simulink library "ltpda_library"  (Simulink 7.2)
settings: Solver=ode45  SolverMode=SingleTasking  StartTime=0.0  StopTime=10.0  RelTol=1e-3
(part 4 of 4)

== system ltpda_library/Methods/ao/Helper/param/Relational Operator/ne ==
  In1 : Inport  OutDataType=sfix(16)  OutScaling=2^0
  ne : M-S-Function  Tag=ne  FunctionName=ltpdasim
  Out1 : Outport  OutDataType=sfix(16)  OutScaling=2^0
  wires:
  In1/1 -> ne/1
  ne/1 -> Out1/1

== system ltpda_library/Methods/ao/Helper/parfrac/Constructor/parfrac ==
  Ground : Ground
  parfrac : M-S-Function  Tag=parfrac  FunctionName=ltpdasim
  Out1 : Outport  OutDataType=sfix(16)  OutScaling=2^0
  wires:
  Ground/1 -> parfrac/1
  parfrac/1 -> Out1/1

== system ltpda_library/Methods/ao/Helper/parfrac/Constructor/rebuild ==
  Ground : Ground
  rebuild : M-S-Function  Tag=rebuild  FunctionName=ltpdasim
  Out1 : Outport  OutDataType=sfix(16)  OutScaling=2^0
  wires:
  Ground/1 -> rebuild/1
  rebuild/1 -> Out1/1

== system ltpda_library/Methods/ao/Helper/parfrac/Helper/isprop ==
  In1 : Inport  OutDataType=sfix(16)  OutScaling=2^0
  isprop : M-S-Function  Tag=isprop  FunctionName=ltpdasim
  Out1 : Outport  OutDataType=sfix(16)  OutScaling=2^0
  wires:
  In1/1 -> isprop/1
  isprop/1 -> Out1/1

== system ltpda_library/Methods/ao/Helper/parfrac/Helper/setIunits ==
  In1 : Inport  OutDataType=sfix(16)  OutScaling=2^0
  setIunits : M-S-Function  Tag=setIunits  FunctionName=ltpdasim
  Out1 : Outport  OutDataType=sfix(16)  OutScaling=2^0
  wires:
  In1/1 -> setIunits/1
  setIunits/1 -> Out1/1

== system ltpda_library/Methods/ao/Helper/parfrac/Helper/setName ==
  In1 : Inport  OutDataType=sfix(16)  OutScaling=2^0
  setName : M-S-Function  Tag=setName  FunctionName=ltpdasim
  Out1 : Outport  OutDataType=sfix(16)  OutScaling=2^0
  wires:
  In1/1 -> setName/1
  setName/1 -> Out1/1

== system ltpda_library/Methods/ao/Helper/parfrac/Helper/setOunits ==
  In1 : Inport  OutDataType=sfix(16)  OutScaling=2^0
  setOunits : M-S-Function  Tag=setOunits  FunctionName=ltpdasim
  Out1 : Outport  OutDataType=sfix(16)  OutScaling=2^0
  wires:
  In1/1 -> setOunits/1
  setOunits/1 -> Out1/1

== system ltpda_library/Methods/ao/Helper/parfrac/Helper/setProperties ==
  In1 : Inport  OutDataType=sfix(16)  OutScaling=2^0
  setProperties : M-S-Function  Tag=setProperties  FunctionName=ltpdasim
  Out1 : Outport  OutDataType=sfix(16)  OutScaling=2^0
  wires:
  In1/1 -> setProperties/1
  setProperties/1 -> Out1/1

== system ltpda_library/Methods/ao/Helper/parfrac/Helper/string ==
  In1 : Inport  OutDataType=sfix(16)  OutScaling=2^0
  string : M-S-Function  Tag=string  FunctionName=ltpdasim
  Out1 : Outport  OutDataType=sfix(16)  OutScaling=2^0
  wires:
  In1/1 -> string/1
  string/1 -> Out1/1

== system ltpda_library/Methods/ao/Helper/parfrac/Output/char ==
  In1 : Inport  OutDataType=sfix(16)  OutScaling=2^0
  Terminator : Terminator
  char : M-S-Function  Tag=char  FunctionName=ltpdasim
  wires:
  char/1 -> Terminator/1
  In1/1 -> char/1

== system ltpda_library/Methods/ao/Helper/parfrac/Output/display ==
  In1 : Inport  OutDataType=sfix(16)  OutScaling=2^0
  Terminator : Terminator
  display : M-S-Function  Tag=display  FunctionName=ltpdasim
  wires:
  display/1 -> Terminator/1
  In1/1 -> display/1

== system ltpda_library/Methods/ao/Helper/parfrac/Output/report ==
  In1 : Inport  OutDataType=sfix(16)  OutScaling=2^0
  Terminator : Terminator
  report : M-S-Function  Tag=report  FunctionName=ltpdasim
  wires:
  report/1 -> Terminator/1
  In1/1 -> report/1

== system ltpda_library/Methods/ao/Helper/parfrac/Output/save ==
  In1 : Inport  OutDataType=sfix(16)  OutScaling=2^0
  Terminator : Terminator
  save : M-S-Function  Tag=save  FunctionName=ltpdasim
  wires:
  save/1 -> Terminator/1
  In1/1 -> save/1

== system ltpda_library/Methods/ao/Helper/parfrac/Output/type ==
  In1 : Inport  OutDataType=sfix(16)  OutScaling=2^0
  Terminator : Terminator
  type : M-S-Function  Tag=type  FunctionName=ltpdasim
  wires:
  type/1 -> Terminator/1
  In1/1 -> type/1

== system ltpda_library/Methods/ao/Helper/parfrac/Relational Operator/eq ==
  In1 : Inport  OutDataType=sfix(16)  OutScaling=2^0
  eq : M-S-Function  Tag=eq  FunctionName=ltpdasim
  Out1 : Outport  OutDataType=sfix(16)  OutScaling=2^0
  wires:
  In1/1 -> eq/1
  eq/1 -> Out1/1

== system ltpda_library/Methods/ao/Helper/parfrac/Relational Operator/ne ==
  In1 : Inport  OutDataType=sfix(16)  OutScaling=2^0
  ne : M-S-Function  Tag=ne  FunctionName=ltpdasim
  Out1 : Outport  OutDataType=sfix(16)  OutScaling=2^0
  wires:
  In1/1 -> ne/1
  ne/1 -> Out1/1

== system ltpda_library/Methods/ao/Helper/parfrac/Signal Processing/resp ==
  In1 : Inport  OutDataType=sfix(16)  OutScaling=2^0
  resp : M-S-Function  Tag=resp  FunctionName=ltpdasim
  Out1 : Outport  OutDataType=sfix(16)  OutScaling=2^0
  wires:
  In1/1 -> resp/1
  resp/1 -> Out1/1

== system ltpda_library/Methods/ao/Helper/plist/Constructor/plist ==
  Ground : Ground
  plist : M-S-Function  Tag=plist  FunctionName=ltpdasim
  Out1 : Outport  OutDataType=sfix(16)  OutScaling=2^0
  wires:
  Ground/1 -> plist/1
  plist/1 -> Out1/1

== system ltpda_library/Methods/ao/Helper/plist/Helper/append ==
  In1 : Inport  OutDataType=sfix(16)  OutScaling=2^0
  append : M-S-Function  Tag=append  FunctionName=ltpdasim
  Out1 : Outport  OutDataType=sfix(16)  OutScaling=2^0
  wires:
  In1/1 -> append/1
  append/1 -> Out1/1

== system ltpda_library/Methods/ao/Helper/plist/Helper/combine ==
  In1 : Inport  OutDataType=sfix(16)  OutScaling=2^0
  combine : M-S-Function  Tag=combine  FunctionName=ltpdasim
  Out1 : Outport  OutDataType=sfix(16)  OutScaling=2^0
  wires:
  In1/1 -> combine/1
  combine/1 -> Out1/1

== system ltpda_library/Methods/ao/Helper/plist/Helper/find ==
  In1 : Inport  OutDataType=sfix(16)  OutScaling=2^0
  find : M-S-Function  Tag=find  FunctionName=ltpdasim
  Out1 : Outport  OutDataType=sfix(16)  OutScaling=2^0
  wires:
  In1/1 -> find/1
  find/1 -> Out1/1

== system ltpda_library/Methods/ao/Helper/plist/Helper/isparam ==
  In1 : Inport  OutDataType=sfix(16)  OutScaling=2^0
  isparam : M-S-Function  Tag=isparam  FunctionName=ltpdasim
  Out1 : Outport  OutDataType=sfix(16)  OutScaling=2^0
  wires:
  In1/1 -> isparam/1
  isparam/1 -> Out1/1

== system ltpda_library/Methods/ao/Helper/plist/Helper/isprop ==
  In1 : Inport  OutDataType=sfix(16)  OutScaling=2^0
  isprop : M-S-Function  Tag=isprop  FunctionName=ltpdasim
  Out1 : Outport  OutDataType=sfix(16)  OutScaling=2^0
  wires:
  In1/1 -> isprop/1
  isprop/1 -> Out1/1

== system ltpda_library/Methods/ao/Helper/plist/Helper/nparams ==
  In1 : Inport  OutDataType=sfix(16)  OutScaling=2^0
  nparams : M-S-Function  Tag=nparams  FunctionName=ltpdasim
  Out1 : Outport  OutDataType=sfix(16)  OutScaling=2^0
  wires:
  In1/1 -> nparams/1
  nparams/1 -> Out1/1

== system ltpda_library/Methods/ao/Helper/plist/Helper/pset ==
  In1 : Inport  OutDataType=sfix(16)  OutScaling=2^0
  pset : M-S-Function  Tag=pset  FunctionName=ltpdasim
  Out1 : Outport  OutDataType=sfix(16)  OutScaling=2^0
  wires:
  In1/1 -> pset/1
  pset/1 -> Out1/1

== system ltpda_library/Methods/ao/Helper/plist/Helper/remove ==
  In1 : Inport  OutDataType=sfix(16)  OutScaling=2^0
  remove : M-S-Function  Tag=remove  FunctionName=ltpdasim
  Out1 : Outport  OutDataType=sfix(16)  OutScaling=2^0
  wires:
  In1/1 -> remove/1
  remove/1 -> Out1/1

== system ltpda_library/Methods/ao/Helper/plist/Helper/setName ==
  In1 : Inport  OutDataType=sfix(16)  OutScaling=2^0
  setName : M-S-Function  Tag=setName  FunctionName=ltpdasim
  Out1 : Outport  OutDataType=sfix(16)  OutScaling=2^0
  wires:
  In1/1 -> setName/1
  setName/1 -> Out1/1

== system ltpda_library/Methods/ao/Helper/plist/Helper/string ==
  In1 : Inport  OutDataType=sfix(16)  OutScaling=2^0
  string : M-S-Function  Tag=string  FunctionName=ltpdasim
  Out1 : Outport  OutDataType=sfix(16)  OutScaling=2^0
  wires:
  In1/1 -> string/1
  string/1 -> Out1/1

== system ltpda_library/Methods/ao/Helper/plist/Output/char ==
  In1 : Inport  OutDataType=sfix(16)  OutScaling=2^0
  Terminator : Terminator
  char : M-S-Function  Tag=char  FunctionName=ltpdasim
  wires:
  char/1 -> Terminator/1
  In1/1 -> char/1

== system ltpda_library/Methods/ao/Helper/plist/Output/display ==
  In1 : Inport  OutDataType=sfix(16)  OutScaling=2^0
  Terminator : Terminator
  display : M-S-Function  Tag=display  FunctionName=ltpdasim
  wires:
  display/1 -> Terminator/1
  In1/1 -> display/1

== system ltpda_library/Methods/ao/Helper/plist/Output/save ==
  In1 : Inport  OutDataType=sfix(16)  OutScaling=2^0
  Terminator : Terminator
  save : M-S-Function  Tag=save  FunctionName=ltpdasim
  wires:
  save/1 -> Terminator/1
  In1/1 -> save/1

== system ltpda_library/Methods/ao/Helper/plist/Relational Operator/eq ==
  In1 : Inport  OutDataType=sfix(16)  OutScaling=2^0
  eq : M-S-Function  Tag=eq  FunctionName=ltpdasim
  Out1 : Outport  OutDataType=sfix(16)  OutScaling=2^0
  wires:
  In1/1 -> eq/1
  eq/1 -> Out1/1

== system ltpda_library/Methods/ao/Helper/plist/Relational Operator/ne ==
  In1 : Inport  OutDataType=sfix(16)  OutScaling=2^0
  ne : M-S-Function  Tag=ne  FunctionName=ltpdasim
  Out1 : Outport  OutDataType=sfix(16)  OutScaling=2^0
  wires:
  In1/1 -> ne/1
  ne/1 -> Out1/1

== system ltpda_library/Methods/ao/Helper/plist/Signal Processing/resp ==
  In1 : Inport  OutDataType=sfix(16)  OutScaling=2^0
  resp : M-S-Function  Tag=resp  FunctionName=ltpdasim
  Out1 : Outport  OutDataType=sfix(16)  OutScaling=2^0
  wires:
  In1/1 -> resp/1
  resp/1 -> Out1/1

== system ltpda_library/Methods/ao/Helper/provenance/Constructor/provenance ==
  Ground : Ground
  provenance : M-S-Function  Tag=provenance  FunctionName=ltpdasim
  Out1 : Outport  OutDataType=sfix(16)  OutScaling=2^0
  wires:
  Ground/1 -> provenance/1
  provenance/1 -> Out1/1

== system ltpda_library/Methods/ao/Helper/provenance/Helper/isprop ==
  In1 : Inport  OutDataType=sfix(16)  OutScaling=2^0
  isprop : M-S-Function  Tag=isprop  FunctionName=ltpdasim
  Out1 : Outport  OutDataType=sfix(16)  OutScaling=2^0
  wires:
  In1/1 -> isprop/1
  isprop/1 -> Out1/1

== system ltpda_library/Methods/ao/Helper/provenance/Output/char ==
  In1 : Inport  OutDataType=sfix(16)  OutScaling=2^0
  Terminator : Terminator
  char : M-S-Function  Tag=char  FunctionName=ltpdasim
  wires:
  char/1 -> Terminator/1
  In1/1 -> char/1

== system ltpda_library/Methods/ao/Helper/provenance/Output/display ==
  In1 : Inport  OutDataType=sfix(16)  OutScaling=2^0
  Terminator : Terminator
  display : M-S-Function  Tag=display  FunctionName=ltpdasim
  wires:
  display/1 -> Terminator/1
  In1/1 -> display/1

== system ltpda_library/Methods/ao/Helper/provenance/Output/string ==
  In1 : Inport  OutDataType=sfix(16)  OutScaling=2^0
  Terminator : Terminator
  string : M-S-Function  Tag=string  FunctionName=ltpdasim
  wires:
  string/1 -> Terminator/1
  In1/1 -> string/1

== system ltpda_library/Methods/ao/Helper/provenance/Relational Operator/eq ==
  In1 : Inport  OutDataType=sfix(16)  OutScaling=2^0
  eq : M-S-Function  Tag=eq  FunctionName=ltpdasim
  Out1 : Outport  OutDataType=sfix(16)  OutScaling=2^0
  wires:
  In1/1 -> eq/1
  eq/1 -> Out1/1

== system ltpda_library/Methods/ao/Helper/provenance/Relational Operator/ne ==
  In1 : Inport  OutDataType=sfix(16)  OutScaling=2^0
  ne : M-S-Function  Tag=ne  FunctionName=ltpdasim
  Out1 : Outport  OutDataType=sfix(16)  OutScaling=2^0
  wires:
  In1/1 -> ne/1
  ne/1 -> Out1/1

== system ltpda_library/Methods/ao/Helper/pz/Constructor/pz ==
  Ground : Ground
  pz : M-S-Function  Tag=pz  FunctionName=ltpdasim
  Out1 : Outport  OutDataType=sfix(16)  OutScaling=2^0
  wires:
  Ground/1 -> pz/1
  pz/1 -> Out1/1

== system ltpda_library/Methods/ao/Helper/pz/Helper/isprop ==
  In1 : Inport  OutDataType=sfix(16)  OutScaling=2^0
  isprop : M-S-Function  Tag=isprop  FunctionName=ltpdasim
  Out1 : Outport  OutDataType=sfix(16)  OutScaling=2^0
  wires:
  In1/1 -> isprop/1
  isprop/1 -> Out1/1

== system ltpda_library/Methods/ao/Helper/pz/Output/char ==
  In1 : Inport  OutDataType=sfix(16)  OutScaling=2^0
  Terminator : Terminator
  char : M-S-Function  Tag=char  FunctionName=ltpdasim
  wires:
  char/1 -> Terminator/1
  In1/1 -> char/1

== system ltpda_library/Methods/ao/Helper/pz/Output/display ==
  In1 : Inport  OutDataType=sfix(16)  OutScaling=2^0
  Terminator : Terminator
  display : M-S-Function  Tag=display  FunctionName=ltpdasim
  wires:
  display/1 -> Terminator/1
  In1/1 -> display/1

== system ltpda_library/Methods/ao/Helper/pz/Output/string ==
  In1 : Inport  OutDataType=sfix(16)  OutScaling=2^0
  Terminator : Terminator
  string : M-S-Function  Tag=string  FunctionName=ltpdasim
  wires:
  string/1 -> Terminator/1
  In1/1 -> string/1

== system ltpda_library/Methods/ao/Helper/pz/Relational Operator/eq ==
  In1 : Inport  OutDataType=sfix(16)  OutScaling=2^0
  eq : M-S-Function  Tag=eq  FunctionName=ltpdasim
  Out1 : Outport  OutDataType=sfix(16)  OutScaling=2^0
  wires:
  In1/1 -> eq/1
  eq/1 -> Out1/1

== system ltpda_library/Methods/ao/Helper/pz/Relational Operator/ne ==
  In1 : Inport  OutDataType=sfix(16)  OutScaling=2^0
  ne : M-S-Function  Tag=ne  FunctionName=ltpdasim
  Out1 : Outport  OutDataType=sfix(16)  OutScaling=2^0
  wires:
  In1/1 -> ne/1
  ne/1 -> Out1/1

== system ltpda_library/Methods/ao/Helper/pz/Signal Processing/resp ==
  In1 : Inport  OutDataType=sfix(16)  OutScaling=2^0
  resp : M-S-Function  Tag=resp  FunctionName=ltpdasim
  Out1 : Outport  OutDataType=sfix(16)  OutScaling=2^0
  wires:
  In1/1 -> resp/1
  resp/1 -> Out1/1

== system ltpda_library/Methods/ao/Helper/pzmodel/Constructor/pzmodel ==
  Ground : Ground
  pzmodel : M-S-Function  Tag=pzmodel  FunctionName=ltpdasim
  Out1 : Outport  OutDataType=sfix(16)  OutScaling=2^0
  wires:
  Ground/1 -> pzmodel/1
  pzmodel/1 -> Out1/1

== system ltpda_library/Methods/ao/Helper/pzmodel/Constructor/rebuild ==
  Ground : Ground
  rebuild : M-S-Function  Tag=rebuild  FunctionName=ltpdasim
  Out1 : Outport  OutDataType=sfix(16)  OutScaling=2^0
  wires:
  Ground/1 -> rebuild/1
  rebuild/1 -> Out1/1

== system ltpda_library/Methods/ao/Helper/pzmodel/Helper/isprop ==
  In1 : Inport  OutDataType=sfix(16)  OutScaling=2^0
  isprop : M-S-Function  Tag=isprop  FunctionName=ltpdasim
  Out1 : Outport  OutDataType=sfix(16)  OutScaling=2^0
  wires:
  In1/1 -> isprop/1
  isprop/1 -> Out1/1

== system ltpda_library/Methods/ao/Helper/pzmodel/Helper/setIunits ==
  In1 : Inport  OutDataType=sfix(16)  OutScaling=2^0
  setIunits : M-S-Function  Tag=setIunits  FunctionName=ltpdasim
  Out1 : Outport  OutDataType=sfix(16)  OutScaling=2^0
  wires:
  In1/1 -> setIunits/1
  setIunits/1 -> Out1/1

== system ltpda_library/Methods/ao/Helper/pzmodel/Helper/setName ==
  In1 : Inport  OutDataType=sfix(16)  OutScaling=2^0
  setName : M-S-Function  Tag=setName  FunctionName=ltpdasim
  Out1 : Outport  OutDataType=sfix(16)  OutScaling=2^0
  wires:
  In1/1 -> setName/1
  setName/1 -> Out1/1

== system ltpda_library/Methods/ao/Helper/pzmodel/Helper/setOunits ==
  In1 : Inport  OutDataType=sfix(16)  OutScaling=2^0
  setOunits : M-S-Function  Tag=setOunits  FunctionName=ltpdasim
  Out1 : Outport  OutDataType=sfix(16)  OutScaling=2^0
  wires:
  In1/1 -> setOunits/1
  setOunits/1 -> Out1/1

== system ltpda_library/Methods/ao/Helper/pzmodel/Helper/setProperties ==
  In1 : Inport  OutDataType=sfix(16)  OutScaling=2^0
  setProperties : M-S-Function  Tag=setProperties  FunctionName=ltpdasim
  Out1 : Outport  OutDataType=sfix(16)  OutScaling=2^0
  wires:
  In1/1 -> setProperties/1
  setProperties/1 -> Out1/1

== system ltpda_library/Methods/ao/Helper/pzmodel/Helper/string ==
  In1 : Inport  OutDataType=sfix(16)  OutScaling=2^0
  string : M-S-Function  Tag=string  FunctionName=ltpdasim
  Out1 : Outport  OutDataType=sfix(16)  OutScaling=2^0
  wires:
  In1/1 -> string/1
  string/1 -> Out1/1

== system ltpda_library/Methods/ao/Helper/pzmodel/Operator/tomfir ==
  In1 : Inport  OutDataType=sfix(16)  OutScaling=2^0
  tomfir : M-S-Function  Tag=tomfir  FunctionName=ltpdasim
  Out1 : Outport  OutDataType=sfix(16)  OutScaling=2^0
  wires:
  In1/1 -> tomfir/1
  tomfir/1 -> Out1/1

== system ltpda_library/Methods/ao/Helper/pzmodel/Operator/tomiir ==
  In1 : Inport  OutDataType=sfix(16)  OutScaling=2^0
  tomiir : M-S-Function  Tag=tomiir  FunctionName=ltpdasim
  Out1 : Outport  OutDataType=sfix(16)  OutScaling=2^0
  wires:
  In1/1 -> tomiir/1
  tomiir/1 -> Out1/1

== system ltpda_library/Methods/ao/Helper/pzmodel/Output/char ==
  In1 : Inport  OutDataType=sfix(16)  OutScaling=2^0
  Terminator : Terminator
  char : M-S-Function  Tag=char  FunctionName=ltpdasim
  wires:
  char/1 -> Terminator/1
  In1/1 -> char/1

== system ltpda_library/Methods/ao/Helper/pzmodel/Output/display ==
  In1 : Inport  OutDataType=sfix(16)  OutScaling=2^0
  Terminator : Terminator
  display : M-S-Function  Tag=display  FunctionName=ltpdasim
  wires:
  display/1 -> Terminator/1
  In1/1 -> display/1

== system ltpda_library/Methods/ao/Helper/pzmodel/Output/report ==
  In1 : Inport  OutDataType=sfix(16)  OutScaling=2^0
  Terminator : Terminator
  report : M-S-Function  Tag=report  FunctionName=ltpdasim
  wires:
  report/1 -> Terminator/1
  In1/1 -> report/1

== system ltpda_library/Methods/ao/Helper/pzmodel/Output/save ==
  In1 : Inport  OutDataType=sfix(16)  OutScaling=2^0
  Terminator : Terminator
  save : M-S-Function  Tag=save  FunctionName=ltpdasim
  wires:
  save/1 -> Terminator/1
  In1/1 -> save/1

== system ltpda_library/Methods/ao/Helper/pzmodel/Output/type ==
  In1 : Inport  OutDataType=sfix(16)  OutScaling=2^0
  Terminator : Terminator
  type : M-S-Function  Tag=type  FunctionName=ltpdasim
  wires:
  type/1 -> Terminator/1
  In1/1 -> type/1

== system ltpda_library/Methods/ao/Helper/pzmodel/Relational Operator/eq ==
  In1 : Inport  OutDataType=sfix(16)  OutScaling=2^0
  eq : M-S-Function  Tag=eq  FunctionName=ltpdasim
  Out1 : Outport  OutDataType=sfix(16)  OutScaling=2^0
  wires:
  In1/1 -> eq/1
  eq/1 -> Out1/1

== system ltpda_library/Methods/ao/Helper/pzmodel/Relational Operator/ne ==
  In1 : Inport  OutDataType=sfix(16)  OutScaling=2^0
  ne : M-S-Function  Tag=ne  FunctionName=ltpdasim
  Out1 : Outport  OutDataType=sfix(16)  OutScaling=2^0
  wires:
  In1/1 -> ne/1
  ne/1 -> Out1/1

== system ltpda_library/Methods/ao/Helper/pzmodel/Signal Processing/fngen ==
  In1 : Inport  OutDataType=sfix(16)  OutScaling=2^0
  fngen : M-S-Function  Tag=fngen  FunctionName=ltpdasim
  Out1 : Outport  OutDataType=sfix(16)  OutScaling=2^0
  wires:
  In1/1 -> fngen/1
  fngen/1 -> Out1/1

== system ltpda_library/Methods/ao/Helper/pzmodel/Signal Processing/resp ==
  In1 : Inport  OutDataType=sfix(16)  OutScaling=2^0
  resp : M-S-Function  Tag=resp  FunctionName=ltpdasim
  Out1 : Outport  OutDataType=sfix(16)  OutScaling=2^0
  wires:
  In1/1 -> resp/1
  resp/1 -> Out1/1

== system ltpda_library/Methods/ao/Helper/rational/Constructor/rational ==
  Ground : Ground
  rational : M-S-Function  Tag=rational  FunctionName=ltpdasim
  Out1 : Outport  OutDataType=sfix(16)  OutScaling=2^0
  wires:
  Ground/1 -> rational/1
  rational/1 -> Out1/1

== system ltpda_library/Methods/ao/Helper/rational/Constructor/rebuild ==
  Ground : Ground
  rebuild : M-S-Function  Tag=rebuild  FunctionName=ltpdasim
  Out1 : Outport  OutDataType=sfix(16)  OutScaling=2^0
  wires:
  Ground/1 -> rebuild/1
  rebuild/1 -> Out1/1

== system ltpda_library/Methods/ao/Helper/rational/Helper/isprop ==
  In1 : Inport  OutDataType=sfix(16)  OutScaling=2^0
  isprop : M-S-Function  Tag=isprop  FunctionName=ltpdasim
  Out1 : Outport  OutDataType=sfix(16)  OutScaling=2^0
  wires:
  In1/1 -> isprop/1
  isprop/1 -> Out1/1

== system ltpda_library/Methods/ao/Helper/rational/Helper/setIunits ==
  In1 : Inport  OutDataType=sfix(16)  OutScaling=2^0
  setIunits : M-S-Function  Tag=setIunits  FunctionName=ltpdasim
  Out1 : Outport  OutDataType=sfix(16)  OutScaling=2^0
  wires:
  In1/1 -> setIunits/1
  setIunits/1 -> Out1/1

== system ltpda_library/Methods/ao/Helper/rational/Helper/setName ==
  In1 : Inport  OutDataType=sfix(16)  OutScaling=2^0
  setName : M-S-Function  Tag=setName  FunctionName=ltpdasim
  Out1 : Outport  OutDataType=sfix(16)  OutScaling=2^0
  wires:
  In1/1 -> setName/1
  setName/1 -> Out1/1

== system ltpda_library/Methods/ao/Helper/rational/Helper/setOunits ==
  In1 : Inport  OutDataType=sfix(16)  OutScaling=2^0
  setOunits : M-S-Function  Tag=setOunits  FunctionName=ltpdasim
  Out1 : Outport  OutDataType=sfix(16)  OutScaling=2^0
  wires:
  In1/1 -> setOunits/1
  setOunits/1 -> Out1/1

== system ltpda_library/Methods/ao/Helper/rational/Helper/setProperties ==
  In1 : Inport  OutDataType=sfix(16)  OutScaling=2^0
  setProperties : M-S-Function  Tag=setProperties  FunctionName=ltpdasim
  Out1 : Outport  OutDataType=sfix(16)  OutScaling=2^0
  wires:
  In1/1 -> setProperties/1
  setProperties/1 -> Out1/1

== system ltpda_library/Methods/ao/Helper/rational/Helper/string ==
  In1 : Inport  OutDataType=sfix(16)  OutScaling=2^0
  string : M-S-Function  Tag=string  FunctionName=ltpdasim
  Out1 : Outport  OutDataType=sfix(16)  OutScaling=2^0
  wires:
  In1/1 -> string/1
  string/1 -> Out1/1

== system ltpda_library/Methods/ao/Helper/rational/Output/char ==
  In1 : Inport  OutDataType=sfix(16)  OutScaling=2^0
  Terminator : Terminator
  char : M-S-Function  Tag=char  FunctionName=ltpdasim
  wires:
  char/1 -> Terminator/1
  In1/1 -> char/1

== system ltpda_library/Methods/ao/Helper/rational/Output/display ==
  In1 : Inport  OutDataType=sfix(16)  OutScaling=2^0
  Terminator : Terminator
  display : M-S-Function  Tag=display  FunctionName=ltpdasim
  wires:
  display/1 -> Terminator/1
  In1/1 -> display/1

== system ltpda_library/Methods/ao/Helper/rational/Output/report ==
  In1 : Inport  OutDataType=sfix(16)  OutScaling=2^0
  Terminator : Terminator
  report : M-S-Function  Tag=report  FunctionName=ltpdasim
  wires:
  report/1 -> Terminator/1
  In1/1 -> report/1

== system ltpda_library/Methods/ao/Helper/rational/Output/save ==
  In1 : Inport  OutDataType=sfix(16)  OutScaling=2^0
  Terminator : Terminator
  save : M-S-Function  Tag=save  FunctionName=ltpdasim
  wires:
  save/1 -> Terminator/1
  In1/1 -> save/1

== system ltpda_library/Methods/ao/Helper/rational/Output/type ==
  In1 : Inport  OutDataType=sfix(16)  OutScaling=2^0
  Terminator : Terminator
  type : M-S-Function  Tag=type  FunctionName=ltpdasim
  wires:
  type/1 -> Terminator/1
  In1/1 -> type/1

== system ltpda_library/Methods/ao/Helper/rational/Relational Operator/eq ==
  In1 : Inport  OutDataType=sfix(16)  OutScaling=2^0
  eq : M-S-Function  Tag=eq  FunctionName=ltpdasim
  Out1 : Outport  OutDataType=sfix(16)  OutScaling=2^0
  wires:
  In1/1 -> eq/1
  eq/1 -> Out1/1

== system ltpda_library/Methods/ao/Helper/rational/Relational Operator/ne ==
  In1 : Inport  OutDataType=sfix(16)  OutScaling=2^0
  ne : M-S-Function  Tag=specwin  Tag=ne  FunctionName=ltpdasim
  Out1 : Outport  OutDataType=sfix(16)  OutScaling=2^0
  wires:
  In1/1 -> ?specwin/1
  ?specwin/1 -> Out1/1

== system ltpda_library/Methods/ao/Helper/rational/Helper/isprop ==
  In1 : Inport  OutDataType=sfix(16)  OutScaling=2^0
  isprop : M-S-Function  Tag=isprop  FunctionName=ltpdasim
  Out1 : Outport  OutDataType=sfix(16)  OutScaling=2^0
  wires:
  In1/1 -> ?ne/1
  ?ne/1 -> Out1/1

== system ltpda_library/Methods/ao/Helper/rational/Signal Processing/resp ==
  In1 : Inport  OutDataType=sfix(16)  OutScaling=2^0
  resp : M-S-Function  Tag=char  Tag=resp  FunctionName=ltpdasim
  Out1 : Outport  OutDataType=sfix(16)  OutScaling=2^0
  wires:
  In1/1 -> resp/1
  resp/1 -> Out1/1

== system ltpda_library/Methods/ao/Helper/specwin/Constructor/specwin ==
  Ground : Ground
  specwin : M-S-Function  Tag=specwin  FunctionName=ltpdasim
  Out1 : Outport  OutDataType=sfix(16)  OutScaling=2^0
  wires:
  Ground/1 -> specwin/1
  specwin/1 -> Out1/1

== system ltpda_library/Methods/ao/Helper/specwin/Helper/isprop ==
  In1 : Inport  OutDataType=sfix(16)  OutScaling=2^0
  In1 : Inport  OutDataType=sfix(16)  OutScaling=2^0
  isprop : M-S-Function  Tag=display  Tag=isprop  FunctionName=ltpdasim
  Out1 : Outport  OutDataType=sfix(16)  OutScaling=2^0
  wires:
  In1/1 -> isprop/1
  isprop/1 -> ?display/1

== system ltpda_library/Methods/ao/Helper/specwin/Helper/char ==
  In1 : Inport  OutDataType=sfix(16)  OutScaling=2^0
  Terminator : Terminator
  char : M-S-Function  Tag=char  FunctionName=ltpdasim
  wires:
  char/1 -> Terminator/1
  In1/1 -> char/1

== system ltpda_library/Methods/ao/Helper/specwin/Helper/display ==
  In1 : Inport  OutDataType=sfix(16)  OutScaling=2^0
  Terminator : Terminator
  plot : M-S-Function  Tag=plot  FunctionName=ltpdasim
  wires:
  plot/1 -> Terminator/1
  In1/1 -> plot/1

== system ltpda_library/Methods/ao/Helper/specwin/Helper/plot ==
  In1 : Inport  OutDataType=sfix(16)  OutScaling=2^0
  Terminator : Terminator
  plot : M-S-Function  Tag=plot  FunctionName=ltpdasim
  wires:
  plot/1 -> Terminator/1
  In1/1 -> plot/1

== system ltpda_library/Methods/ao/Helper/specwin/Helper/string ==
  In1 : Inport  OutDataType=sfix(16)  OutScaling=2^0
  Terminator : Terminator
  string : M-S-Function  Tag=string  FunctionName=ltpdasim
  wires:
  string/1 -> Terminator/1
  In1/1 -> string/1

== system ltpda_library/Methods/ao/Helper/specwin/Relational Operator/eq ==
  In1 : Inport  OutDataType=sfix(16)  OutScaling=2^0
  eq : M-S-Function  Tag=eq  FunctionName=ltpdasim
  Out1 : Outport  OutDataType=sfix(16)  OutScaling=2^0
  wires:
  In1/1 -> eq/1
  eq/1 -> Out1/1

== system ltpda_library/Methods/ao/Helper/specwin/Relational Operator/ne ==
  In1 : Inport  OutDataType=sfix(16)  OutScaling=2^0
  ne : M-S-Function  Tag=ne  FunctionName=ltpdasim
  Out1 : Outport  OutDataType=sfix(16)  OutScaling=2^0
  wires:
  In1/1 -> ne/1
  ne/1 -> Out1/1

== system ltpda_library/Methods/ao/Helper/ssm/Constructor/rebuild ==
  Ground : Ground
  rebuild : M-S-Function  Tag=rebuild  FunctionName=ltpdasim
  Out1 : Outport  Tag=rebuild  FunctionName=ltpdasim  OutDataType=sfix(16)  OutScaling=2^0
  Out1 : Outport  OutDataType=sfix(16)  OutScaling=2^0
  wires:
  Ground/1 -> rebuild/1
  rebuild/1 -> Out1/1

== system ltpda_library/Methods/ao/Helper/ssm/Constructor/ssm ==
  Ground : Ground
  ssm : M-S-Function  Tag=ssm  FunctionName=ltpdasim
  Out1 : Outport  OutDataType=sfix(16)  OutScaling=2^0
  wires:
  Ground/1 -> ssm/1
  ssm/1 -> Out1/1

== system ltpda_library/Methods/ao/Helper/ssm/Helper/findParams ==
  In1 : Inport  OutDataType=sfix(16)  OutScaling=2^0
  findParams : M-S-Function  Tag=findParams  FunctionName=ltpdasim
  Out1 : Outport  OutDataType=sfix(16)  OutScaling=2^0
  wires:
  In1/1 -> findParams/1
  findParams/1 -> Out1/1

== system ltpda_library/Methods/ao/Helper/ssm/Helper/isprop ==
  In1 : Inport  OutDataType=sfix(16)  OutScaling=2^0
  isprop : M-S-Function  Tag=isprop  FunctionName=ltpdasim
  Out1 : Outport  OutDataType=sfix(16)  OutScaling=2^0
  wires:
  In1/1 -> isprop/1
  isprop/1 -> Out1/1
